TYPE ST_EcMasterDevState :
STRUCT
	eEcState	 		: E_EcCommState;
	nReserved			: ARRAY [0..2] OF UINT;

	bLinkError			: BOOL;
	bResetRequired		: BOOL;
	bMissFrmRedMode		: BOOL;
	bWatchdogTriggerd	: BOOL;
	bDriverNotFound		: BOOL;
	bResetActive		: BOOL;
	bAtLeastOneNotInOp	: BOOL;
	bDcNotInSync		: BOOL;
END_STRUCT
END_TYPE
